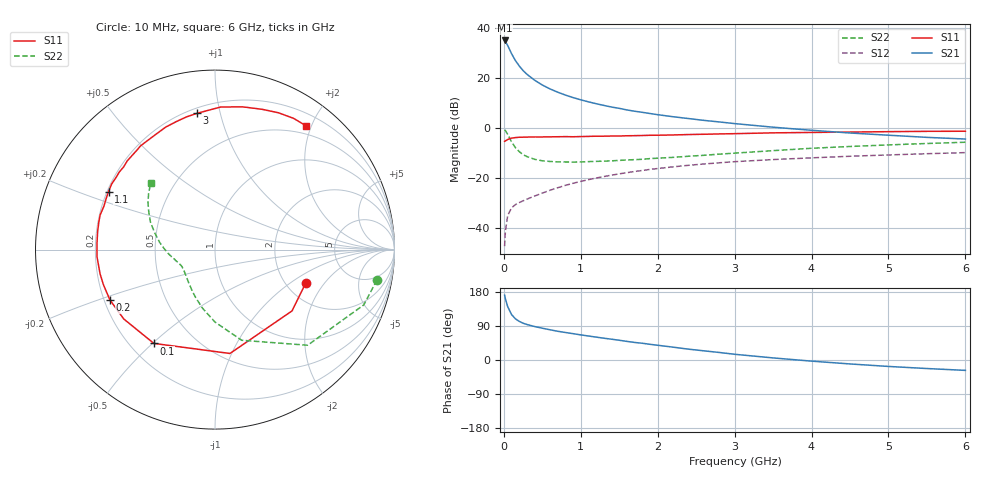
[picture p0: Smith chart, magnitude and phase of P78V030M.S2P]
! SIEMENS Small Signal Semiconductors
! BFP196
! Si NPN RF Bipolar Junction Transistor in SOT143
! VCE = 8 V  IC = 30 mA
! Common Emitter S-Parameters:  May  1996
# GHz  S  MA  R  50
!  f  S11  S21  S12  S22
! GHz  MAG  ANG  MAG  ANG  MAG  ANG  MAG  ANG
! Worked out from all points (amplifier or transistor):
!   36 points, 10 MHz to 6 GHz, reference 50 ohm
!   highest |S21| = 35.0 dB at 10 MHz (marker M1)
!   |S21| within 3 dB of that: start of sweep to 65.27 MHz
!   unconditionally stable (mu >= 1): 615.5 MHz to 4.528 GHz
!   at 250 MHz: K = 0.68, MSG = 26.1 dB, |S12| = -29.2 dB
!   at 1.4 GHz: K = 1.09, MAG = 11.8 dB, |S12| = -18.9 dB
!   at 6 GHz: K = 0.97, MSG = 2.7 dB, |S12| = -9.9 dB
!   lowest NFmin = 1.40 dB at 500 MHz
!   S11 on the Smith chart (normalised r, x): 10 MHz: 2.56, -1.33; 100 MHz: 0.29, -0.50; 200 MHz: 0.22, -0.22; 1.1 GHz: 0.21, +0.24; 3 GHz: 0.23, +0.85; 6 GHz: 0.37, +1.93
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0.01  0.539 -19.9  56.09 171.0  0.0043 81.8  0.9182 -10.6
0.02  0.5485 -38.5  53.36 161.6  0.0085 72.8  0.8843 -20.4
0.05  0.5847 -81.8  44.52 140.8  0.0176 59.1  0.742 -45.9
0.1  0.6239 -123.1  30.6 120.0  0.0251 47.6  0.5267 -73.6
0.15  0.6387 -142.8  22.26 108.8  0.0291 43.3  0.4036 -90.0
0.2  0.6492 -154.4  17.37 101.9  0.032 43.9  0.3348 -101.8
0.25  0.6518 -162.6  14.02 97.1  0.0347 45.5  0.2911 -111.2
0.3  0.6543 -168.1  11.82 93.7  0.0375 47.3  0.2669 -117.8
0.4  0.6588 -176.7  8.995 88.3  0.0433 50.6  0.2351 -128.7
0.5  0.6584 177.4  7.199 83.9  0.0495 52.8  0.2197 -136.5
0.6  0.6611 171.7  6.017 79.8  0.0565 54.4  0.2128 -141.9
0.7  0.6648 167.1  5.179 75.8  0.0634 55.3  0.2089 -145.9
0.9  0.6644 158.7  4.037 69.5  0.0779 55.8  0.207 -152.4
1.1  0.6753 151.4  3.316 63.3  0.0921 55.6  0.2113 -156.6
1.3  0.6821 143.9  2.814 57.5  0.1064 53.9  0.2159 -160.4
1.6  0.695 134.8  2.285 49.1  0.1271 51.2  0.2283 -164.8
2.2  0.7213 117.4  1.671 33.9  0.1662 44.0  0.2573 -174.1
3  0.7659 97.5  1.218 15.1  0.2106 33.3  0.3121 172.3
3.5  0.7952 87.7  1.032 5.5  0.2324 26.8  0.3506 164.1
4.5  0.8244 71.5  0.79 -10.4  0.2704 15.4  0.4243 150.4
5.5  0.8523 59.1  0.646 -22.5  0.3041 4.9  0.4872 139.3
6  0.8566 53.5  0.598 -27.4  0.3199 -0.8  0.516 133.8
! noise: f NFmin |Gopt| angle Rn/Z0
0.5  1.4  0.4  -173  0.08
0.9  1.6  0.5  -166  0.08
1.5  2.4  0.61  -150  0.14
2  2.9  0.71  -129  0.2
